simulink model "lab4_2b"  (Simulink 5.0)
settings: Solver=FixedStepDiscrete  StartTime=0.0  StopTime=10*1e-3  FixedStep=T  RelTol=1e-3
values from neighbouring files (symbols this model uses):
  T = 1/Fsamp    (= 0.0001)    [lab4_4.m]

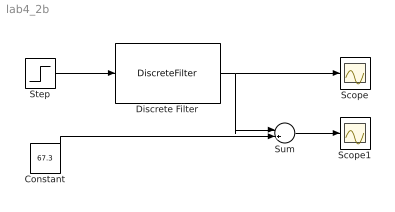
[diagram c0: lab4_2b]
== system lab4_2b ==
  Constant : Constant  Value=67.3
  Discrete Filter : DiscreteFilter  Numerator="[2  1]"  Denominator="[1  -1.8*cos(pi/16)  0.81]"  SampleTime=T
  Scope : Scope
  Scope1 : Scope
  Step : Step  Time=0  SampleTime=0
  Sum : Sum  Inputs=|++
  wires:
  Discrete Filter/1 -> Scope/1, Sum/1
  Step/1 -> Discrete Filter/1
  Constant/1 -> Sum/2
  Sum/1 -> Scope1/1
